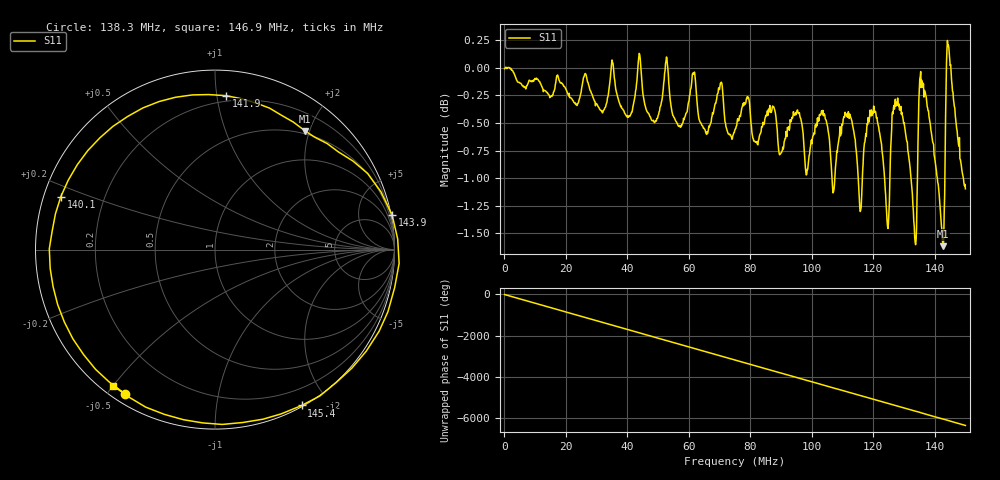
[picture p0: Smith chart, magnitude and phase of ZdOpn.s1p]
# MHz S RI R 400.0
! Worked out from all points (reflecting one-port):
!   1000 points, 100 kHz to 150 MHz, reference 400 ohm
!   lowest |S11| = -1.6 dB at 142.8 MHz (marker M1), VSWR 10.79, Z = 182 + j773 ohm
!   phase of S11 starts at -4 deg and turns -6375 deg over the sweep
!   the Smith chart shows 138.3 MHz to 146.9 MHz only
!   S11 on the Smith chart (normalised r, x): 138.3 MHz: 0.04, -0.55; 140.1 MHz: 0.05, +0.17; 141.9 MHz: 0.16, +1.06; 143.9 MHz: -0, +10; 145.4 MHz: 0.01, -1.70; 146.9 MHz: 0.03, -0.50
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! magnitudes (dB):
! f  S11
! 100 kHz  0.0
! 18.85 MHz  -0.1
! 37.6 MHz  -0.3
! 49.15 MHz  -0.5
! 52.75 MHz  0.1
! 56.35 MHz  -0.5
! 61.6 MHz  -0.1
! 75.15 MHz  -0.6
! 93.9 MHz  -0.4
! 98.55 MHz  -0.9
! 104 MHz  -0.4
! 107.1 MHz  -1.1
! 112.7 MHz  -0.4
! 115.8 MHz  -1.3
! 119.7 MHz  -0.4
! 124.5 MHz  -1.4
! 126.9 MHz  -0.4
! 131.4 MHz  -0.8
! 133.5 MHz  -1.5
! 135.6 MHz  -0.2
! 138.3 MHz  -0.5
! 140.1 MHz  -0.8
! 141.9 MHz  -1.3
! 142.8 MHz  -1.6
! 143.9 MHz  0.0
! 145.4 MHz  -0.1
! 146.9 MHz  -0.5
! 150 MHz  -1.1
